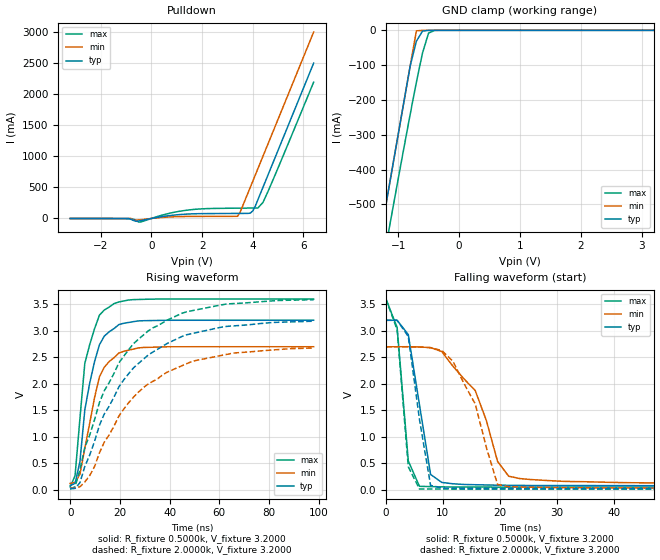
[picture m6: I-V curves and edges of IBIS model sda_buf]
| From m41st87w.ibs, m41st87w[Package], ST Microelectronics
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|   Model sda_buf
[Model]   sda_buf
Model_type   I/O_open_drain
Polarity   Non-Inverting
Enable   Active-High
Vinl =   1.5000V
Vinh =   3.5000V
Vmeas =   1.5000V
Cref =  50.0000pF
Rref =   1.0000k
Vref =   1.7500V
C_comp   3.2900pF   3.2200pF   4.6400pF
[Temperature Range]   27.0000   85.0000   -40.0000
[Voltage Range]   3.2000V   2.7000V   3.6000V
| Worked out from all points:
|   slope of the pulldown table from 0 to 0.48 V, typ, clamps not added: 14.3 ohm
|   GND clamp passes 1 mA (typ) near -0.54 V on its own axis
|   rising waveform, R_fixture 0.5000k, V_fixture 3.2000: 20-80 % time 6.5ns typ, 7.03ns min, 5.97ns max; typ from 0.081 V to 3.2 V
|   rising waveform, R_fixture 2.0000k, V_fixture 3.2000: 20-80 % time 23.8ns typ, 25.8ns min, 22.7ns max; typ from 0.019 V to 3.18 V
|   falling waveform, R_fixture 0.5000k, V_fixture 3.2000: 20-80 % time 2.78ns typ, 6.37ns min, 1.66ns max; typ from 3.2 V to 0.079 V
|   falling waveform, R_fixture 2.0000k, V_fixture 3.2000: 20-80 % time 2.61ns typ, 5.33ns min, 1.63ns max; typ from 3.2 V to 0.02 V
[Pulldown]
| voltage   I(typ)   I(min)   I(max)
-3.2V     0A         0A         -700uA
-900mV    0A         0A         -5.54mA
-500mV    -39.83mA   -23.28mA   -59.76mA
1.3V      68.19mA    31.87mA    127.7mA
3.4V      81.17mA    34.99mA    165.9mA
3.5V      81.34mA    100mA      166.2mA
3.9V      85.33mA    500mA      167.5mA
4V        121.5mA    600mA      167.8mA
4.2V      300mA      800mA      168.7mA
4.4V      500mA      1A         256.9mA
5V        1.1A       1.6A       816.8mA
6.4V      2.5A       3A         2.194A
[GND_clamp]
| voltage   I(typ)   I(min)   I(max)
-3.2V     -2.5A      -2.5A      -2.591A
-1.3V     -600mA     -600mA     -717.2mA
-1.2V     -500mA     -500mA     -620.1mA
-1.1V     -400mA     -400mA     -523.5mA
-800mV    -100.6mA   -100mA     -239.3mA
-700mV    -31.18mA   -1.472mA   -148.9mA
-600mV    -2.147mA   -113.6uA   -65.37mA
-500mV    -71.61uA   -15.45uA   -7.938mA
-400mV    -3.348uA   -2.557uA   -84.18uA
3.2V      -7.457nA   1.819uA    83.17pA
[Ramp]
| variable   typ   min   max
dV/dt_r   1.8834/7.9164n   1.5647/8.6940n   2.1365/7.4557n
dV/dt_f   1.8831/2.3164n   1.5648/6.0689n   2.1362/1.4189n
R_load = 0.6450k
[Rising Waveform]
R_fixture = 0.5000k
V_fixture = 3.2000
V_fixture_min = 2.7000
V_fixture_max = 3.6000
| time   V(typ)   V(min)   V(max)
0s        81mV       120.4mV    54.24mV
1.96ns    121.2mV    137.5mV    266.1mV
3.92ns    531.1mV    292.8mV    1.346V
5.88ns    1.506V     781.8mV    2.386V
9.8ns     2.419V     1.739V     3.04V
11.76ns   2.736V     2.131V     3.295V
13.72ns   2.901V     2.313V     3.393V
19.6ns    3.119V     2.581V     3.546V
27.44ns   3.188V     2.678V     3.592V
98ns      3.2V       2.7V       3.6V
[Rising Waveform]
R_fixture = 2.0000k
V_fixture = 3.2000
V_fixture_min = 2.7000
V_fixture_max = 3.6000
| time   V(typ)   V(min)   V(max)
0s        19.01mV    29.26mV    11.95mV
1.96ns    26.13mV    32.1mV     60.12mV
3.92ns    134.3mV    57.45mV    374mV
5.88ns    441.3mV    148.3mV    800.2mV
9.8ns     914mV      438.2mV    1.321V
13.72ns   1.431V     899.5mV    1.871V
21.56ns   2.075V     1.524V     2.521V
31.36ns   2.542V     1.997V     2.998V
50.96ns   2.968V     2.444V     3.398V
98ns      3.182V     2.676V     3.587V
[Falling Waveform]
R_fixture = 0.5000k
V_fixture = 3.2000
V_fixture_min = 2.7000
V_fixture_max = 3.6000
| time   V(typ)   V(min)   V(max)
0s        3.2V       2.7V       3.601V
1.96ns    3.2V       2.7V       3.066V
3.92ns    2.931V     2.701V     546mV
5.88ns    1.61V      2.696V     65.98mV
7.84ns    289.8mV    2.686V     60.32mV
9.8ns     139.4mV    2.61V      55.81mV
15.68ns   95.86mV    1.874V     51.35mV
19.6ns    87.07mV    537.1mV    50.97mV
21.56ns   85mV       256.3mV    50.63mV
98ns      79.16mV    118.8mV    51.06mV
[Falling Waveform]
R_fixture = 2.0000k
V_fixture = 3.2000
V_fixture_min = 2.7000
V_fixture_max = 3.6000
| time   V(typ)   V(min)   V(max)
0s        3.2V       2.7V       3.601V
1.96ns    3.2V       2.7V       3.023V
3.92ns    2.894V     2.701V     434.6mV
5.88ns    1.331V     2.696V     16.51mV
7.84ns    82.99mV    2.683V     15.46mV
9.8ns     34.13mV    2.63V      14.58mV
11.76ns   28.56mV    2.428V     12.79mV
15.68ns   24.24mV    1.621V     12.87mV
19.6ns    22.42mV    101.9mV    13.08mV
98ns      20.37mV    29.7mV     13.3mV
